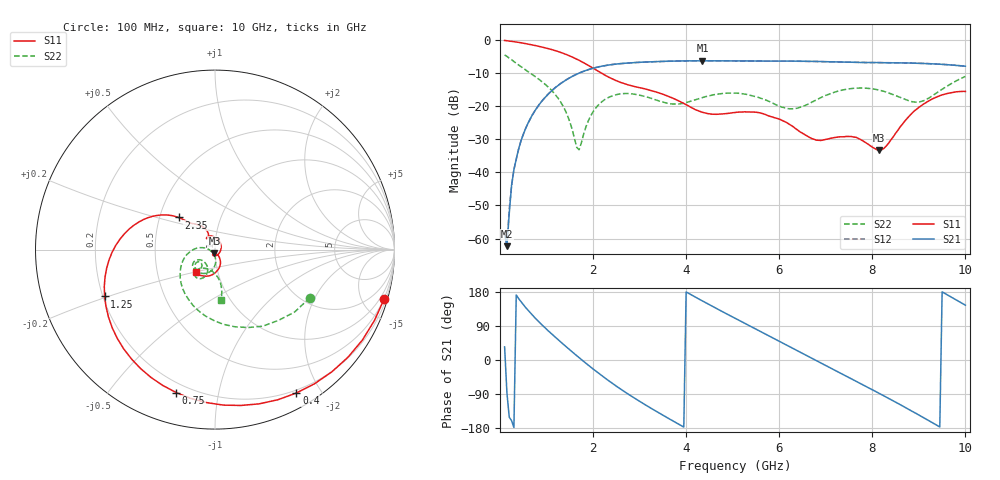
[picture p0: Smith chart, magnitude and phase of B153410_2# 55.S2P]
!  2-Port S-parameters saved by WinCal
! VAR MeasName=S-Parameters (CALIBRATED_DATA) read from VNA (N5245A)
! VAR MeasDate=2016-12-23 10:02:16
! VAR NAME=B153410_2# 55
! VAR FILENAME=B153410_2# 55.S2P
! VAR DATE=2016-12-23 10:02:16
! VAR PHYS_PORTS=1,2
# Hz S DB R 50
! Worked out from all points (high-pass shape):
!   199 points, 100 MHz to 10 GHz, reference 50 ohm
!   highest |S21| = -6.29 dB at 4.35 GHz (marker M1); lowest = -62.3 dB at 150 MHz (marker M2)
!   |S21| within 3 dB of the highest: 1.831 GHz to end of sweep
!   lowest |S11| = -33.4 dB at 8.15 GHz (marker M3), VSWR 1.04, Z = 49.6 - j2.11 ohm
!   |S11| at or under -10 dB: 2.177 GHz to end of sweep
!   |S22| runs from -33.2 to -4.5 dB; largest |S21 - S12| = 0.0024
!   S11 on the Smith chart (normalised r, x): 100 MHz: 0.45, -7.00; 400 MHz: 0.17, -1.70; 750 MHz: 0.15, -0.75; 1.25 GHz: 0.21, -0.20; 2.35 GHz: 0.63, +0.24; 10 GHz: 0.78, -0.21
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1e8  -0.16 -16.2  -58.61 34.7  -57.78 26.2  -4.54 -26.9
1.5e8  -0.24 -23.9  -62.31 -87.0  -61.74 -68.2  -4.98 -38.1
2.5e8  -0.42 -39.0  -43.85 -160.0  -44.09 -158.2  -5.98 -58.1
4e8  -0.74 -60.5  -33.00 162.3  -33.11 163.1  -7.56 -83.7
7.5e8  -1.67 -105.2  -21.41 111.5  -21.43 112.0  -10.99 -129.7
1.25e9  -3.50 -157.0  -13.74 53.4  -13.71 53.3  -17.61 -177.5
1.5e9  -4.83 -178.5  -11.43 26.8  -11.40 26.7  -24.68 170.7
1.65e9  -5.80 170.1  -10.34 11.3  -10.32 11.2  -32.46 -158.7
1.75e9  -6.52 163.3  -9.73 1.1  -9.71 1.0  -31.06 -103.4
2e9  -8.53 149.5  -8.54 -23.6  -8.55 -23.8  -21.72 -88.9
2.35e9  -11.34 138.6  -7.54 -55.9  -7.55 -56.1  -17.26 -108.3
2.85e9  -13.94 132.6  -6.89 -97.4  -6.88 -97.5  -16.32 -134.0
3.4e9  -15.93 122.0  -6.53 -138.5  -6.54 -138.5  -18.36 -144.8
4.35e9  -21.86 117.9  -6.29 155.9  -6.31 155.8  -17.41 -127.5
5.05e9  -21.94 125.6  -6.33 110.0  -6.35 110.1  -16.06 -140.7
5.85e9  -23.26 91.4  -6.39 59.1  -6.39 59.2  -19.02 -149.3
6.7e9  -29.79 -1.0  -6.47 4.6  -6.49 4.6  -18.81 -110.9
7.65e9  -29.41 -111.5  -6.77 -56.2  -6.77 -56.0  -14.56 -120.5
8.15e9  -33.35 -98.2  -6.85 -88.3  -6.86 -88.1  -15.16 -130.2
8.35e9  -31.21 -69.8  -6.91 -101.3  -6.89 -101.1  -15.98 -131.2
9e9  -20.37 -73.4  -7.04 -145.1  -7.03 -145.1  -18.79 -105.5
1e10  -15.56 -130.1  -7.94 144.6  -7.94 144.6  -11.03 -83.1
